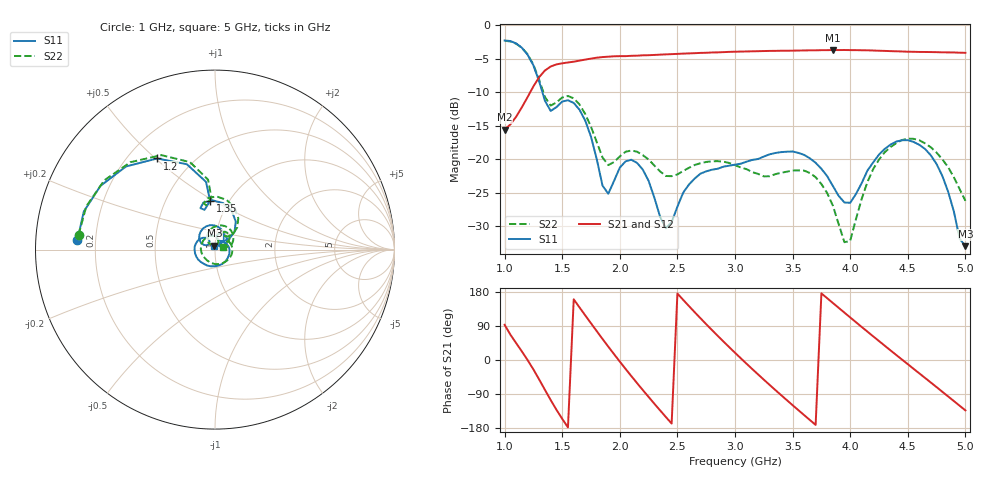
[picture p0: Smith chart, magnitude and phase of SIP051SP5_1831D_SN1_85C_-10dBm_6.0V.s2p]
# GHz  S  dB  R  50
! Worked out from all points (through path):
!   81 points, 1 GHz to 5 GHz, reference 50 ohm
!   highest |S21| = -3.71 dB at 3.85 GHz (marker M1); lowest = -15.6 dB at 1 GHz (marker M2)
!   lowest |S11| = -33.0 dB at 5 GHz (marker M3), VSWR 1.05, Z = 49.6 + j2.2 ohm
!   |S11| at or under -10 dB: 1.328 GHz to end of sweep
!   |S22| runs from -32.4 to -2.3 dB; largest |S21 - S12| = 0.0022
!   S11 on the Smith chart (normalised r, x): 1 GHz: 0.13, +0.03; 1.2 GHz: 0.32, +0.51; 1.35 GHz: 0.82, +0.48; 5 GHz: 0.99, +0.04
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1  -2.28 176.2  -15.57 92.9  -15.57 93.0  -2.33 173.9
1.2  -4.42 122.4  -10.71 -0.4  -10.71 -0.4  -4.36 119.6
1.35  -11.27 95.7  -6.76 -78.7  -6.75 -78.7  -10.71 94.0
1.55  -11.20 93.3  -5.56 -177.9  -5.55 -178.0  -10.56 88.4
1.7  -14.23 53.4  -5.14 117.7  -5.12 117.7  -13.25 53.3
1.9  -25.14 70.3  -4.70 35.3  -4.68 35.4  -20.86 57.0
2  -21.24 79.8  -4.62 -4.2  -4.61 -4.2  -19.57 65.2
2.2  -21.55 35.7  -4.50 -79.4  -4.51 -79.3  -19.39 41.1
2.35  -28.59 23.0  -4.40 -133.0  -4.38 -133.0  -21.82 32.9
2.5  -27.09 55.2  -4.29 175.4  -4.26 175.4  -22.26 36.0
2.7  -22.14 12.1  -4.14 110.3  -4.12 110.2  -20.59 19.2
2.85  -21.41 -34.2  -4.06 63.8  -4.04 63.8  -20.28 -8.3
3  -20.80 -77.0  -3.96 19.1  -3.95 19.1  -20.87 -43.9
3.15  -20.09 -116.0  -3.90 -23.9  -3.90 -23.9  -21.91 -90.7
3.35  -19.06 -159.5  -3.83 -79.2  -3.83 -79.2  -22.22 -167.0
3.7  -20.52 135.6  -3.75 -171.3  -3.74 -171.3  -22.67 91.0
3.85  -23.99 121.8  -3.71 150.3  -3.70 150.3  -26.93 65.6
4  -26.49 144.6  -3.72 112.3  -3.72 112.3  -32.16 114.3
4.15  -21.68 155.5  -3.75 74.7  -3.75 74.7  -23.38 127.6
4.35  -17.81 128.0  -3.87 25.4  -3.88 25.5  -18.18 95.9
4.7  -19.41 65.3  -4.01 -59.5  -4.01 -59.5  -18.21 33.2
5  -32.95 99.7  -4.12 -133.0  -4.12 -133.1  -26.19 16.6
